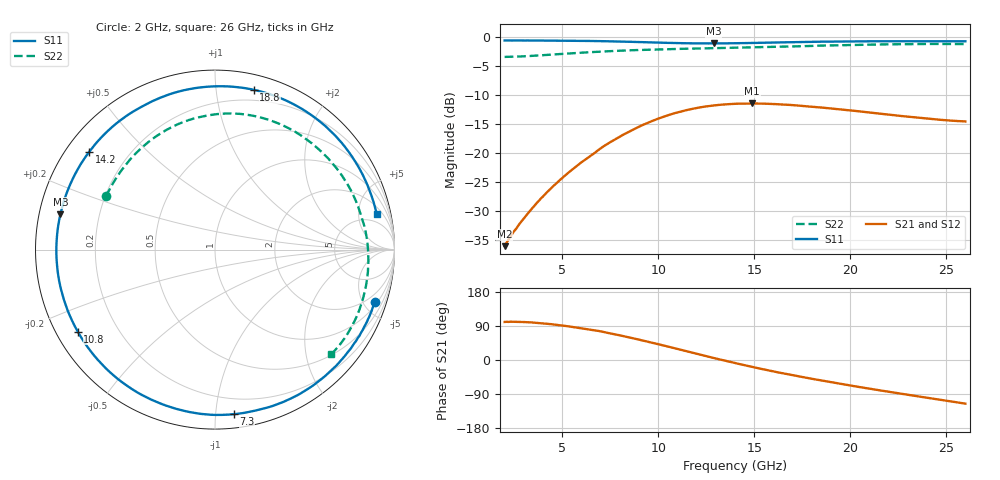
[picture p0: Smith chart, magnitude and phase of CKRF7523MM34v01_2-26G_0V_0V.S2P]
! CHUO DENSHI KOGYO Co.,Ltd.
! 8. March 2017
! CKRF7523MM34_RT5880
! N-channel HJ-FET
! Vds = 0V Vgs = 0V
# Hz S  MA  R 50
!	f	S11	S21	S12	S22
!	Hz	MAG	ANG	MAG	ANG	MAG	ANG	MAG	ANG
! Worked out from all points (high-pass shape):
!   241 points, 2 GHz to 26 GHz, reference 50 ohm
!   highest |S21| = -11.46 dB at 14.9 GHz (marker M1); lowest = -36.1 dB at 2 GHz (marker M2)
!   |S21| within 3 dB of the highest: 9.707 GHz to 25.39 GHz (15.68 GHz wide, 89.4 % of centre)
!   lowest |S11| = -1.1 dB at 12.9 GHz (marker M3), VSWR 16.17, Z = 3.13 + j5.61 ohm
!   |S11| at or under -10 dB: nowhere
!   |S22| runs from -3.4 to -1.2 dB; largest |S21 - S12| = 0.00053
!   S11 on the Smith chart (normalised r, x): 2 GHz: 1.23, -5.96; 7.3 GHz: 0.09, -1.12; 10.8 GHz: 0.06, -0.27; 14.2 GHz: 0.07, +0.34; 18.8 GHz: 0.11, +1.26; 26 GHz: 3.10, +8.10
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2e9  0.9374 -18.3  0.01559 100.3  0.01572 100.8  0.6754 153.9
2.8e9  0.9364 -26.5  0.02462 100.4  0.02463 100.5  0.6812 141.9
4.1e9  0.9349 -40.6  0.04369 96.2  0.04391 96.5  0.701 124.4
6e9  0.9302 -64.4  0.08276 83.6  0.08274 83.6  0.7349 102.2
7.3e9  0.9228 -83.5  0.1179 72.4  0.1179 72.4  0.755 89.1
8e9  0.9187 -95.1  0.1382 65.0  0.1383 64.9  0.7646 82.6
8.7e9  0.9111 -107.5  0.1591 57.2  0.1592 57.3  0.7726 76.4
9.3e9  0.9055 -118.8  0.1772 50.2  0.1773 50.3  0.7782 71.3
1e10  0.8985 -132.7  0.1976 41.7  0.1978 41.7  0.7843 65.7
1.08e10  0.8908 -149.2  0.2188 31.7  0.2189 31.7  0.7903 59.4
1.18e10  0.8853 -170.2  0.2406 19.0  0.2407 19.0  0.7967 52.0
1.29e10  0.8835 167.1  0.257 5.2  0.2571 5.2  0.8041 44.3
1.4e10  0.8869 145.9  0.2656 -8.1  0.2655 -8.0  0.812 36.6
1.42e10  0.8877 142.3  0.2661 -10.4  0.2664 -10.4  0.8134 35.2
1.49e10  0.8916 130.0  0.2673 -18.3  0.2674 -18.3  0.8186 30.4
1.64e10  0.9014 106.8  0.2622 -34.2  0.2625 -34.2  0.8296 20.2
1.8e10  0.912 85.8  0.2503 -49.6  0.2506 -49.6  0.8415 9.4
1.88e10  0.9162 76.4  0.244 -56.8  0.2442 -56.8  0.8483 3.9
2.04e10  0.9213 59.4  0.2292 -70.6  0.2293 -70.6  0.8597 -6.9
2.2e10  0.9229 44.4  0.214 -83.8  0.2144 -83.8  0.868 -17.4
2.39e10  0.9226 28.4  0.1984 -98.8  0.1986 -98.8  0.8741 -29.3
2.6e10  0.9217 12.3  0.1868 -115.2  0.187 -115.2  0.8719 -42.0
